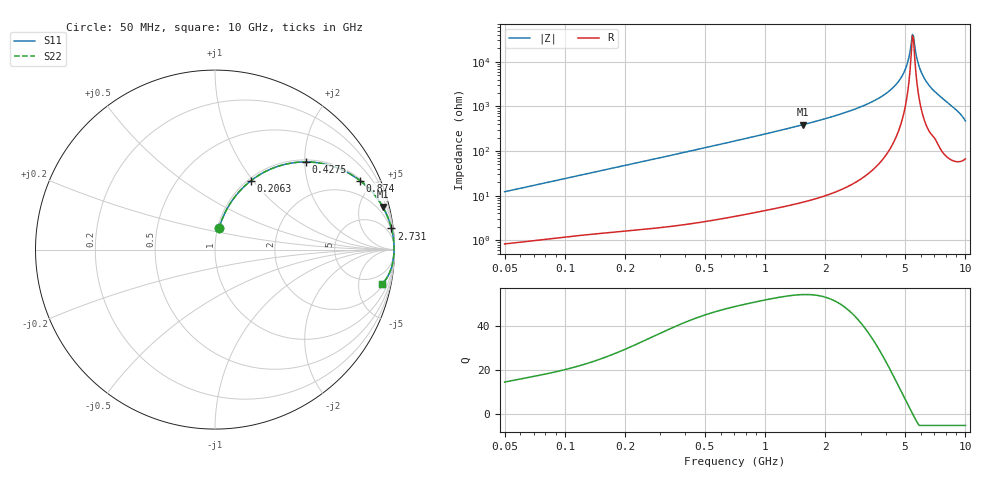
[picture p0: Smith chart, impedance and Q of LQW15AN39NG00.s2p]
!Murata Part Number: LQW15AN39NG00
!These Parameters are Measured in Series Mode Connection
!  o--[Z]--o
!Port1  Port2
!  o-------o
!Freq. Start=50[MHz] Stop=10[GHz], 401[Steps]
# Hz S RI R 50
!Freq.(Hz)	S 11(Real)	S 11(Imag)	S 21(Real)	S 21(Imag)	S 12(Real)	S 12(Imag)	S 22(Real)	S 22(Imag)
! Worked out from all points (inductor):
!   401 points, 50 MHz to 10 GHz, reference 50 ohm
!   read as one part in series: L = 38.6 nH near 51.34 MHz
!   highest Q = 54.4 at 1.545 GHz (marker M1), where L = 40 nH
!   self-resonance near 5.437 GHz
!   S11 on the Smith chart (normalised r, x): 50 MHz: 1.02, +0.24; 206.3 MHz: 1.03, +0.98; 427.5 MHz: 1.05, +2.02; 874 MHz: 1.08, +4.18; 2.731 GHz: 1, +17; 10 GHz: 2.33, -9.35
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5e7  0.0225 0.1183  0.9775 -0.1183  0.9775 -0.1183  0.0225 0.1183
1.214486e8  0.0879 0.2617  0.9121 -0.2617  0.9121 -0.2617  0.0879 0.2617
2.062982e8  0.2013 0.3847  0.7987 -0.3847  0.7987 -0.3847  0.2013 0.3847
2.949953e8  0.3321 0.4575  0.6679 -0.4575  0.6679 -0.4575  0.3321 0.4575
4.274518e8  0.5055 0.4885  0.4945 -0.4885  0.4945 -0.4885  0.5055 0.4885
7.071068e8  0.7347 0.4314  0.2653 -0.4314  0.2653 -0.4314  0.7347 0.4314
8.740297e8  0.8094 0.3831  0.1906 -0.3831  0.1906 -0.3831  0.8094 0.3831
1.544852e9  0.934 0.2393  0.066 -0.2393  0.066 -0.2393  0.934 0.2393
1.717543e9  0.9473 0.2144  0.0527 -0.2144  0.0527 -0.2144  0.9473 0.2144
2.730534e9  0.9832 0.1181  0.0168 -0.1181  0.0168 -0.1181  0.9832 0.1181
3.511936e9  0.9923 0.0734  0.00768 -0.0734  0.00768 -0.0734  0.9923 0.0734
4.171863e9  0.9959 0.0447  0.00414 -0.0447  0.00414 -0.0447  0.9959 0.0447
4.577181e9  0.997 0.0295  0.003 -0.0295  0.003 -0.0295  0.997 0.0295
4.890587e9  0.9975 0.0186  0.00251 -0.0186  0.00251 -0.0186  0.9975 0.0186
5.156693e9  0.9977 0.00979  0.0023 -0.00979  0.0023 -0.00979  0.9977 0.00979
5.365732e9  0.9977 0.00312  0.00227 -0.00312  0.00227 -0.00312  0.9977 0.00312
5.509778e9  0.9977 -0.00137  0.0023 0.00137  0.0023 0.00137  0.9977 -0.00137
5.583245e9  0.9977 -0.00364  0.00234 0.00364  0.00234 0.00364  0.9977 -0.00364
5.88704e9  0.9974 -0.0129  0.00263 0.0129  0.00263 0.0129  0.9974 -0.0129
6.125686e9  0.997 -0.02  0.00302 0.02  0.00302 0.02  0.997 -0.02
6.458996e9  0.9961 -0.0298  0.00388 0.0298  0.00388 0.0298  0.9961 -0.0298
1e10  0.9324 -0.1897  0.0676 0.1897  0.0676 0.1897  0.9324 -0.1897
